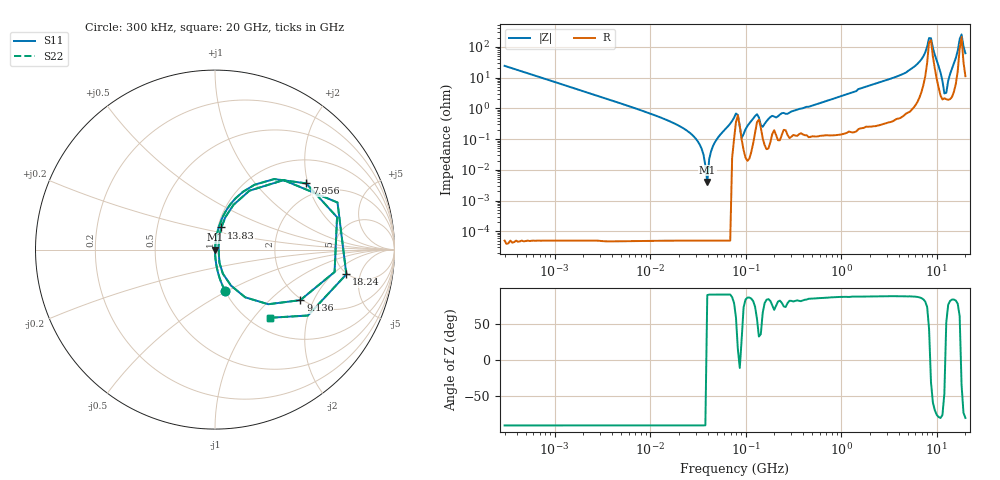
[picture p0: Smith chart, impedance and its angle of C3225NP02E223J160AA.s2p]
! S-parameter Generated by TDK Corporation
! Copyright(C) 2015 TDK Corporation.
! All Rights Reserved.
! TDK P/N: C3225NP02E223J160AA (Multilayer Ceramic Chip Capacitors)
! Property: C=22nF
! Size(LxWxT): 3.2x2.5x1.6mm, 0.126x0.098x0.063inches
! Model Type: s2p (Touchstone File Format Version 1.0)
! Frequency: DC=Yes Start=0.3MHz Stop=20000MHz 243points Log-sweep
! Note:
! Model Generated on Jun. 23, 2015
! Hash(MD5):
! Port Assignments:
!  1 ---| |--- 2
! Applicable Conditions:
!  Temperature = 25 degC
!  DC Bias Voltage = 0 V
!  Small Signal Operation
! Terms and conditions regarding TDK Simulation Models
! (1)This simulation model is being provided solely for informational purposes. Please refer to the specifications of the products in terms of detailed characteristics of such products.
! (2)In no event shall TDK Corporation of any of its subsidiaries be liable for any loss or damage arising, directly or indirectly,
!  From any information contained in this simulation model, including, but not limited to loss or damages arising from any inaccuracies, omissions or errors in connection with such information.
! (3)Any and all copyrights on this simulation model are owned by TDK Corporation.
!  Duplication or redistribution of this simulation model without prior written permission from TDK Corporation is prohibited.
! (4)This simulation model is subject to any modification or change without any prior notice.
! (5)Neither TDK Corporation nor any of its subsidiaries shall make any warranty, express or implied,
!  Including but not limited to the correctness, implied warranties of merchantability and fitness for a particular purpose with respect to this simulation models.
! (6)The use of this simulation model shall be deemed to have consented to the terms and conditions hereof.
# MHz S MA R 50
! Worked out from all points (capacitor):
!   242 points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, 300 kHz to 20 GHz, reference 50 ohm
!   read as one part in series: C = 21.9 nF near 314.2 kHz
!   lowest |Z| = 4.08 mohm at 39.7 MHz (marker M1)
!   series resonance near 39.3 MHz, so ESL is about 750 pH
!   S11 on the Smith chart (normalised r, x): 300 kHz: 1.00, -0.48; 7.956 GHz: 1.60, +1.95; 9.136 GHz: 1.96, -1.59; 13.83 GHz: 1.04, +0.26; 18.24 GHz: 4.90, -3.03; 20 GHz: 1.22, -1.22
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0.3  0.2349 -76.4  0.972 13.6  0.972 13.6  0.2349 -76.4
1.985118  0.0364 -87.9  0.9993 2.1  0.9993 2.1  0.0364 -87.9
12.54397  0.005224 -91.5  0.9998 0.3  0.9998 0.3  0.005224 -91.5
28.7559  0.001223 -98.0  0.9998 0.1  0.9998 0.1  0.001223 -98.0
39.70457  0.0001659 165.8  0.9998 -0.0  0.9998 -0.0  0.0001659 165.8
47.74252  0.0008056 100.6  0.9999 -0.0  0.9999 -0.0  0.0008056 100.6
79.26541  0.006795 58.6  0.9964 -0.3  0.9964 -0.3  0.006795 58.6
91.01907  0.001111 30.6  0.999 -0.0  0.999 -0.0  0.001111 30.6
131.6019  0.00641 56.1  0.9964 -0.3  0.9964 -0.3  0.00641 56.1
151.1161  0.002521 64.9  0.9989 -0.1  0.9989 -0.1  0.002521 64.9
500.8786  0.01239 83.6  0.9987 -0.7  0.9987 -0.7  0.01239 83.6
3165.055  0.08774 82.7  0.9926 -5.0  0.9926 -5.0  0.08774 82.7
6318.653  0.2687 71.1  0.9476 -15.6  0.9476 -15.6  0.2687 71.1
7956.199  0.6278 36.0  0.614 -36.8  0.614 -36.8  0.6278 36.0
8724.45  0.6778 -10.6  0.3547 19.8  0.3547 19.8  0.6778 -10.6
9135.962  0.5525 -30.6  0.5941 28.0  0.5941 28.0  0.5525 -30.6
10985.48  0.1409 -71.9  0.9648 8.0  0.9648 8.0  0.1409 -71.9
12046.24  0.02975 -44.4  0.979 1.3  0.979 1.3  0.02975 -44.4
13832.49  0.1285 74.0  0.9724 -7.3  0.9724 -7.3  0.1285 74.0
16632.79  0.5438 45.4  0.7257 -32.0  0.7257 -32.0  0.5438 45.4
18238.85  0.7447 -10.7  0.2933 24.0  0.2933 24.0  0.7447 -10.7
20000  0.4894 -50.9  0.7887 28.8  0.7887 28.8  0.4894 -50.9
